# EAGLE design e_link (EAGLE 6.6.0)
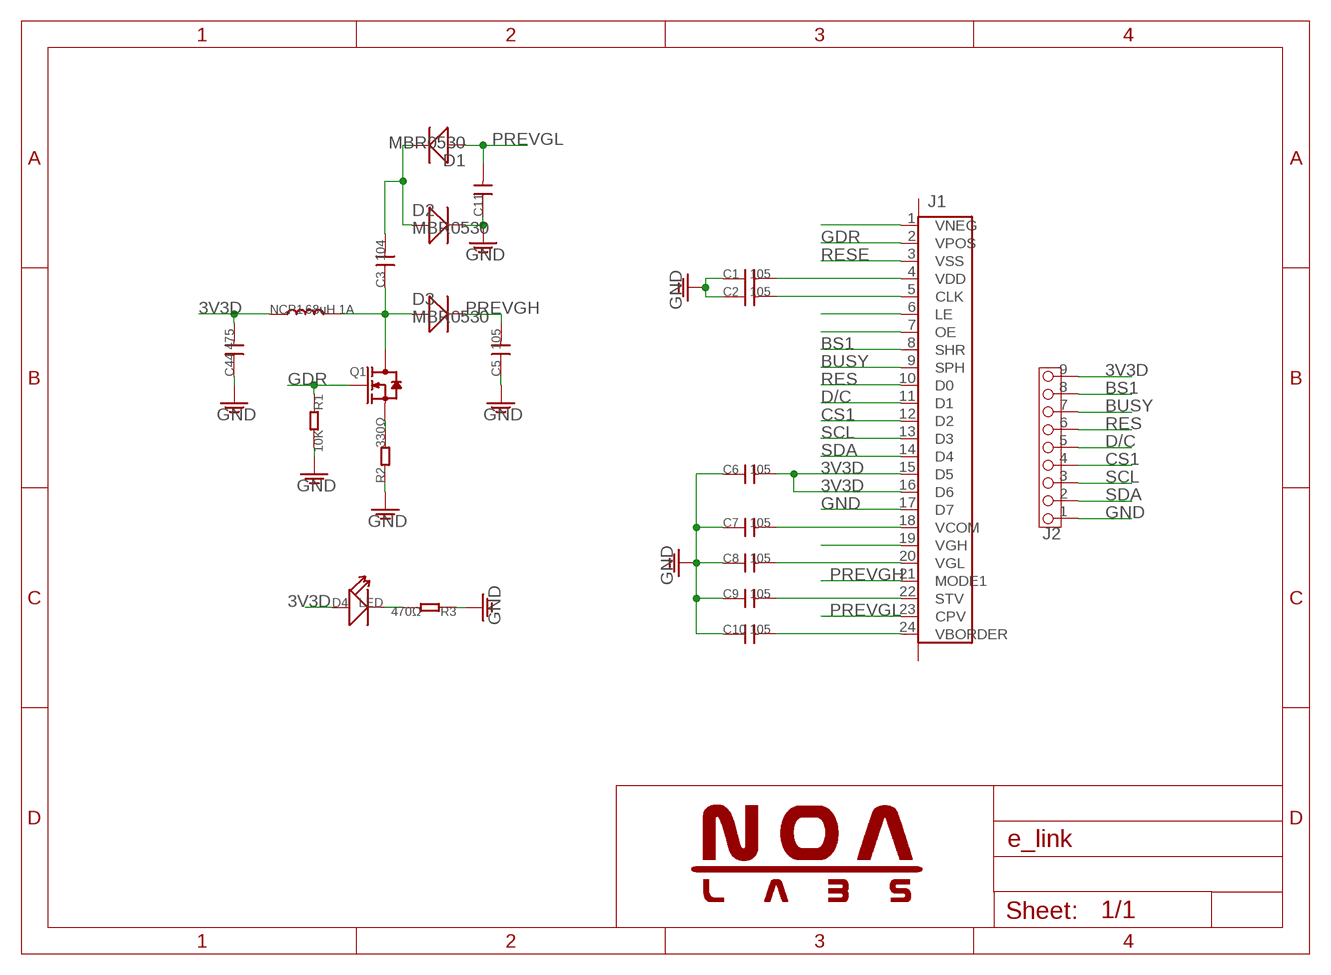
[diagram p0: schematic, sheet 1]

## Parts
C1  105  C-0603  [0603]
C2  105  C-0603  [0603]
C3  104  C-0603  [0603]
C5  105  C-0603  [0603]
C6  105  C-0603  [0603]
C7  105  C-0603  [0603]
C8  105  C-0603  [0603]
C9  105  C-0603  [0603]
C10  105  C-0603  [0603]
C11  C-0603  [0603]
C44  475  C-0603  [0603]
D1  MBR0530  RS1M  [SOD123]
D2  MBR0530  RS1M  [SOD123]
D3  MBR0530  RS1M  [SOD123]
D4  LED  LED'0603'  [LED-0603]
J1  FPC-24P-0.5PFC24/0.5MM上接  [24P-0.5-1]
J2  SMD2.549P  [SMD2.54*9P]
NCP1  68uH 1A  NCP1  [GDNR5040]
Q1  SI1304BDL_1  [SOT323]
R1  10K  R-0603  [0603]
R2  330Ω  R-0603  [0603]
R3  470Ω  R-0603  [0603]

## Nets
3V3D: C6.2 C44.2 D4.+ J1.15(D5) J1.16(D6) J2.9 NCP1.1
BS1: J1.8(SHR) J2.8
BUSY: J1.9(SPH) J2.7
CS1: J1.12(D2) J2.4
D/C: J1.11(D1) J2.5
GDR: J1.2(VPOS) Q1.1 R1.1
GND: C1.1 C2.1 C5.1 C6.1 C7.1 C8.1 C9.1 C10.1 C11.1 C44.1 D2.- J1.17(D7) J2.1 R1.2 R2.1 R3.1
N$1: J1.1(VNEG)
N$2: D4.- R3.2
N$4: C1.2 J1.4(VDD)
N$5: C2.2 J1.5(CLK)
N$6: J1.6(LE)
N$7: J1.7(OE)
N$9: C3.1 D3.+ NCP1.2 Q1.3
N$10: C3.2 D1.- D2.+
N$18: C7.2 J1.18(VCOM)
N$19: J1.19(VGH)
N$20: C8.2 J1.20(VGL)
N$22: C9.2 J1.22(STV)
N$24: C10.2 J1.24(VBORDER)
PREVGH: C5.2 D3.- J1.21(MODE1)
PREVGL: C11.2 D1.+ J1.23(CPV)
RES: J1.10(D0) J2.6
RESE: J1.3(VSS) Q1.2 R2.2
SCL: J1.13(D3) J2.3
SDA: J1.14(D4) J2.2
Unconnected: J1.25 J1.26

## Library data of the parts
C1-C3 C5-C11 C44 = Discrete:C*: Ceramic Capacitors
D1-D3 = Discrete:RS1M: RS1M SOD123
D4 = Discretex:LED*
J1 = Connector:FPC-24P-0.5: PFC24/0.5MM上接
J2 = Connector:SMD2.54*9P: SMD2.54*9P
NCP1 = Discrete:NCP1
Q1 = Discrete:SI1304BDL_1
R1-R3 = Discrete:R*

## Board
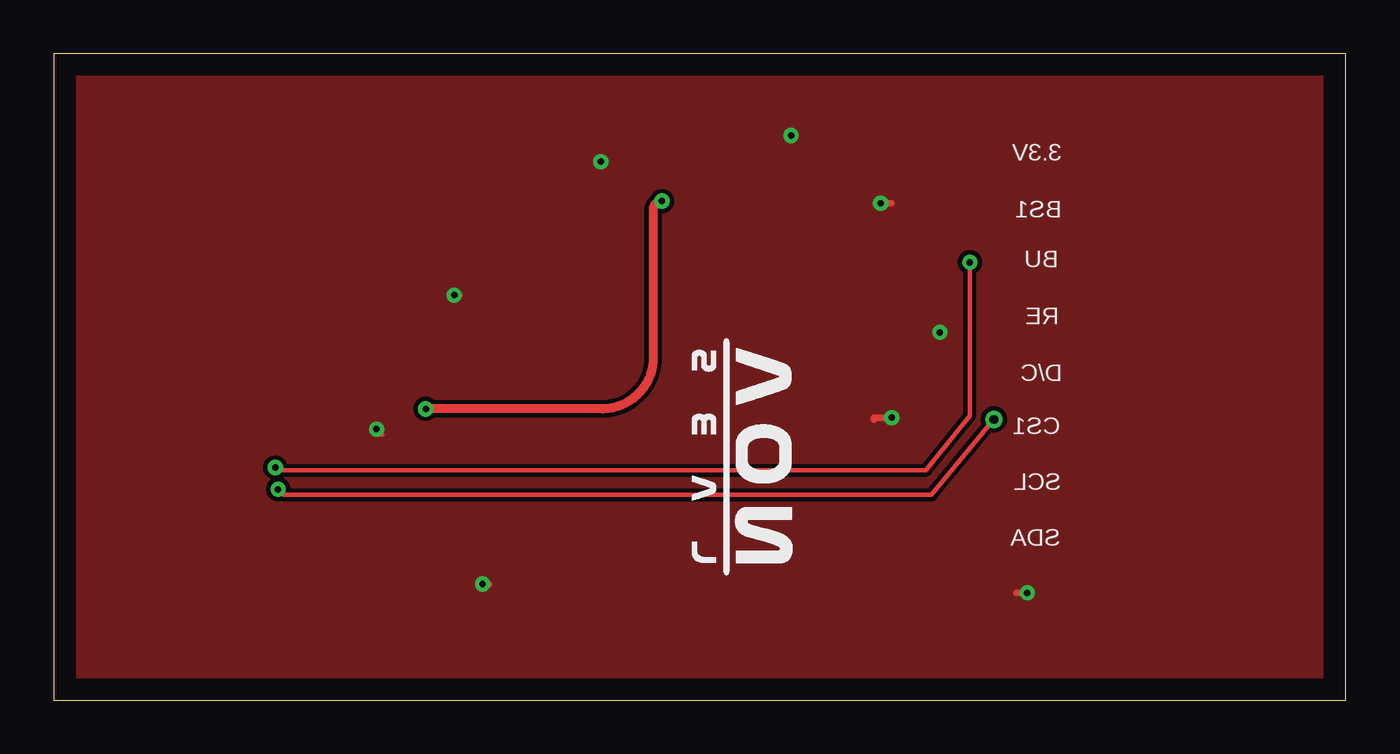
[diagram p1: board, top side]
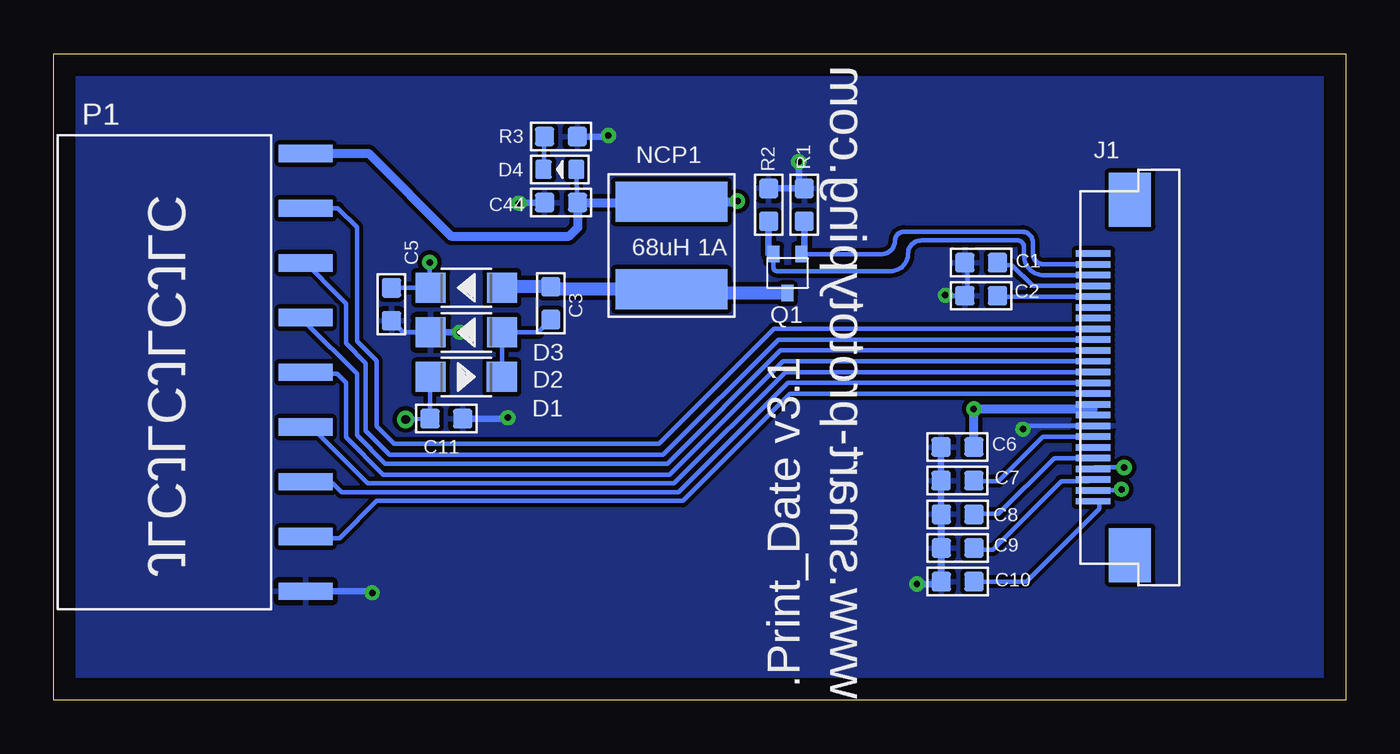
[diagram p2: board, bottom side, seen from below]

Size 60 x 30 mm. Coordinates in mm from the lower left corner, seen from the top.
Outline: 0,0 60,0 60,30 0,30 0,0
Copper layers (1*16): Top 0.035mm / dielectric 1.5mm / Bottom 0.035mm
Design rules "default": minimum track width 10mil, minimum drill 0.6mm, track to track 8mil, track to pad 8mil, pad to pad 8mil, via to via 8mil, smd to smd 8mil, copper to edge 40mil, drill to drill 8mil, minimum pad ring 10mil, minimum via ring 8mil, stop-mask expansion 4mil, vias tented up to drill 0mil, thermal gap 10mil

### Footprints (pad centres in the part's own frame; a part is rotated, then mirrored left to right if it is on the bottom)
0603 = smd 0.889 x 0.889: 1 -0.762,0; 2 0.762,0
SOD123 = smd 1.397 x 1.397: + 1.651,0; - -1.651,0
LED-0603 = smd 0.762 x 0.889: + -0.762,0; - 0.762,0
24P-0.5-1 = smd 1.6 x 0.3: 1 0,6.5; 2 0,6; 3 0,5.5; 4 0,5; 5 0,4.5; 6 0,4; 7 0,3.5; 8 0,3; 9 0,2.5; 10 0,2; 11 0,1.5; 12 0,1; 13 0,0.5; 14 0,0; 15 0,-0.5; 16 0,-1; 17 0,-1.5; 18 0,-2; 19 0,-2.5; 20 0,-3; 21 0,-3.5; 22 0,-4; 23 0,-4.5; 24 0,-5 | smd 1.95 x 2.5: 25 1.7,-7.5; 26 1.7,9
SMD2.54*9P = smd 2.5 x 0.8: 1 0,10.16; 2 0,7.62; 3 0,5.08; 4 0,2.54; 5 0,0; 6 0,-2.54; 7 0,-5.08; 8 0,-7.62; 9 0,-10.16
GDNR5040 = smd 5.2 x 1.85: 1 -0.127,2.032; 2 -0.127,-2.032
SOT323 = smd 0.559 x 0.762: 1 0,0; 2 1.3,0; 3 0.655,1.81

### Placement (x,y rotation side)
C1  16.93,20.31 0 bottom
C2  16.93,18.77 0 bottom
C3  36.92,18.42 270 bottom
C5  44.32,18.37 90 bottom
C6  18.03,11.75 0 bottom
C7  18.03,10.19 0 bottom
C8  18.02,8.62 0 bottom
C9  18.02,7.06 0 bottom
C10  18.02,5.5 0 bottom
C11  41.77,13.06 180 bottom
C44  36.44,23.1 0 bottom
D1  40.84,15 180 bottom
D2  40.84,17.07 0 bottom
D3  40.84,19.14 0 bottom
D4  36.5,24.63 180 bottom
J1  11.72,14.23 0 bottom
J2  48.31,15.21 180 bottom
NCP1  31.19,21.1 0 bottom
Q1  25.27,20.7 180 bottom
R1  25.15,22.99 90 bottom
R2  26.8,22.99 270 bottom
R3  36.45,26.16 180 bottom

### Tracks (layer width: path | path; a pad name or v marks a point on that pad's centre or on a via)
3V3D  (via drill 0.3)
  Top 0.406: v28.25,23.16 arc90 27.84,22.76 27.84,15.95 arc-90 25.5,13.51 v17.27,13.51
  Bottom 0.203: C44.2 D4.+
  Bottom 0.305: C6.2 arc-90 C6.2 | J1.16 11.72,13.51 J1.15
  Bottom 0.406: J2.9 45.39,25.37 41.55,21.54 36.07,21.54 35.66,21.95 35.66,23.08 | 35.66,23.08 C44.2 | 35.66,23.08 31.37,23.08 NCP1.1 28.28,23.13 v28.25,23.16 | 11.72,13.51 v17.27,13.51 C6.2
BS1
  Bottom 0.203: J1.8 26.56,17.23 31.9,11.89 44.2,11.89 45.01,12.7 45.01,15.75 45.92,16.66 45.92,21.95 46.81,22.83 J2.8
BUSY
  Bottom 0.203: J1.9 26.35,16.73 31.7,11.38 44.4,11.38 45.52,12.5 45.52,15.65 46.43,16.56 46.43,18.39 46.74,18.69 J2.7
CS1
  Bottom 0.203: J1.12 26.02,15.23 31.19,10.06 45.41,10.06 48.03,12.67 J2.4
D/C
  Bottom 0.203: J1.11 26.13,15.73 31.39,10.46 44.7,10.46 46.43,12.19 46.43,14.73 46.84,15.14 48.23,15.14 J2.5
GDR
  Bottom 0.203: Q1.1 21.57,20.7 arc-90 20.93,21.34 arc90 20.52,21.74 15.04,21.74 arc90 14.53,21.23 14.53,20.73 arc-90 14.03,20.23 J1.2
  Bottom 0.305: R1.1 25.15,20.7 Q1.1
GND  (via drill 0.3)
  Top 0.203: v14.99,12.57 15.24,12.32 | v18.59,18.8 18.9,18.8
  Top 0.305: v19.91,5.38 20.22,5.38 | v45.21,4.98 44.7,4.98 | v38.91,13.11 38.1,13.11 38.1,13.01 | v41.15,17.07 41.15,16.97 | v34.24,26.21 34.04,26.21 | v38.41,23.06 38.91,23.06 | v25.4,24.99 25.6,24.99
  Bottom 0.203: J1.17 14.83,12.73 v14.99,12.57 | C1.1 arc90 17.58,20.19 17.58,18.8 arc90 17.61,18.77 C2.1 18.56,18.77 arc90 v18.59,18.8 | D2.- 43.78,17.07 C5.1
  Bottom 0.305: C10.1 C9.1 C8.1 18.79,8.62 C7.1 C6.1 18.8,5.38 v19.91,5.38 | J2.1 45.21,5.05 v45.21,4.98 | C11.1 38.91,13.06 v38.91,13.11 | D2.- v41.15,17.07 | R3.1 34.24,26.16 v34.24,26.21 | C44.1 38.41,23.1 v38.41,23.06 | R2.1 R1.2 25.4,23.75 v25.4,24.99
  pour Top: 0,0 59.99,0 59.99,0.03 59.99,30 0,30
  pour Bottom: 0,0 59.99,0 59.99,0.03 59.99,30 0,30
N$2
  Bottom 0.203: D4.- R3.2
N$4
  Bottom 0.203: J1.4 14.53,19.23 15.49,20.19 16.05,20.19 C1.2
N$5
  Bottom 0.203: J1.5 16.13,18.73 C2.2
N$9
  Bottom 0.61: Q1.3 31.14,18.89 arc90 NCP1.2 36.8,19.07 arc90 C3.1 39.15,19.18 arc-90 D3.+
N$10
  Bottom 0.203: D1.- D2.+ 37.51,17.07 C3.2
N$18
  Bottom 0.203: J1.18 14.06,12.23 16.13,10.16 17.24,10.16 C7.2
N$20
  Bottom 0.203: J1.20 13.54,11.23 16.13,8.64 17.24,8.64 C8.2
N$22
  Bottom 0.203: J1.22 11.87,10.23 11.94,10.16 13.21,10.16 16.38,6.99 17.19,6.99 C9.2
N$24
  Bottom 0.203: J1.24 11.43,9.23 11.43,8.89 14.82,5.5 C10.2
PREVGH  (via drill 0.3)
  Top 0.203: v42.55,20.32 42.55,13.21 40.51,10.67 10.41,10.67 v10.29,10.79
  Bottom 0.203: v42.55,20.32 42.55,19.19 D3.- C5.2 | v10.29,10.79 11.65,10.79 J1.21
PREVGL  (via drill 0.3, 0.4)
  Top 0.203: v10.41,9.78 10.67,9.53 40.77,9.53 v43.66,13.03
  Bottom 0.203: J1.23 10.47,9.73 v10.41,9.78 | v43.66,13.03 42.55,13.05 C11.2 42.53,14.96 D1.+
RES
  Bottom 0.203: J1.10 26.24,16.23 31.5,10.97 44.6,10.97 45.92,12.29 45.92,15.14 48.31,17.52 J2.6 48.23,17.68
RESE
  Bottom 0.203: Q1.2 26.57,20.07 arc-90 26.42,19.91 21.13,19.91 arc-90 20.32,20.73 arc90 19.71,21.34 15.24,21.34 arc90 14.94,21.03 14.94,20.62 arc-90 14.04,19.73 J1.3
  Bottom 0.305: R2.2 26.8,20.7 Q1.2
SCL
  Bottom 0.203: J1.13 25.91,14.73 30.99,9.65 46.63,9.65 47.04,10.06 48.23,10.06 J2.3
SDA
  Bottom 0.203: J1.14 25.8,14.23 30.79,9.25 45.01,9.25 46.74,7.52 48.23,7.52 J2.2

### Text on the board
tPlace: 3.3V | BS1 | BU | RE | D/C | CS1 | SCL | SDA
bPlace: www.smart-prototyping.com | P1 | .Print_Date v3.1
bNames: JLCJLCJLCJLC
